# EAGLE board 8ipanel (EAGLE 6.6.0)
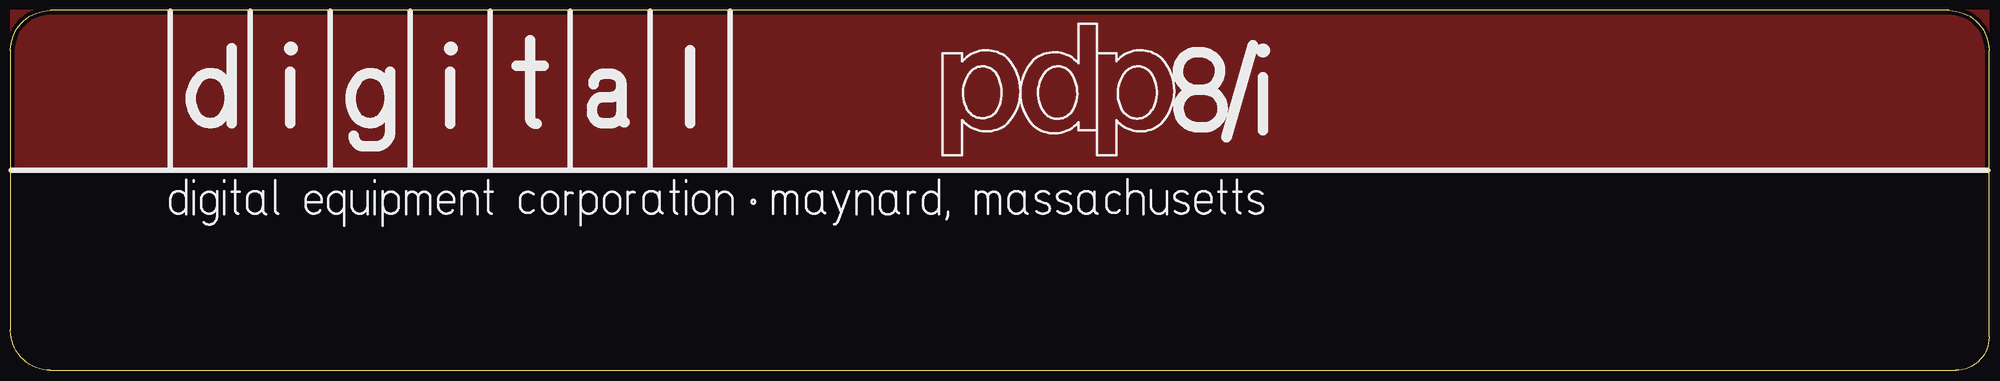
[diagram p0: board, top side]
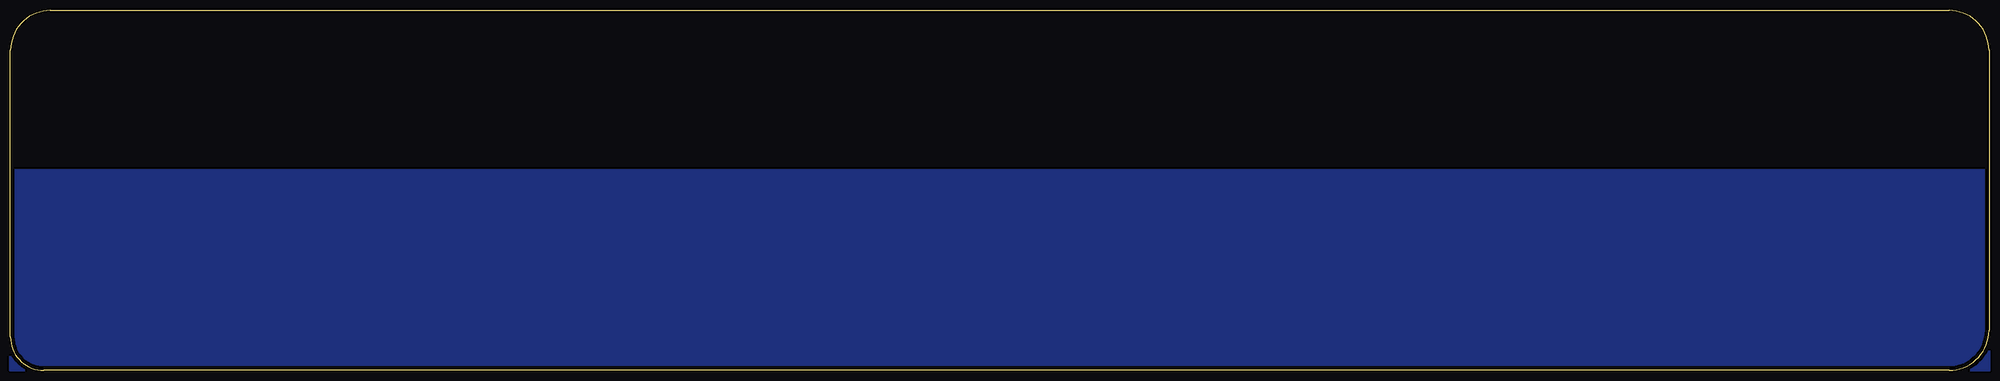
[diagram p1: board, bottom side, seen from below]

Size 471.49 x 85.72 mm. Coordinates in mm from the lower left corner, seen from the top.
Outline: 9.53,0 463.55,0 arc90 471.49,7.94 471.49,76.2 arc90 461.96,85.72 9.53,85.72 arc90 0,76.2 0,9.53 arc90 9.53,0
Copper layers (1*16): Top 0.035mm / dielectric 1.5mm / Bottom 0.035mm
Design rules "default": minimum track width 10mil, minimum drill 24mil, track to track 8mil, track to pad 8mil, pad to pad 8mil, via to via 8mil, smd to smd 8mil, copper to edge 40mil, drill to drill 8mil, minimum pad ring 10mil, minimum via ring 8mil, stop-mask expansion 4mil, vias tented up to drill 0mil, thermal gap 10mil

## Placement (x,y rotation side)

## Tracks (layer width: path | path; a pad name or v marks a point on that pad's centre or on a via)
S$1
  pour Top: 0,47.62 471.49,47.62 471.49,85.72 0,85.72
S$2
  pour Bottom: 0,47.62 0,0 471.49,0 471.49,47.62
